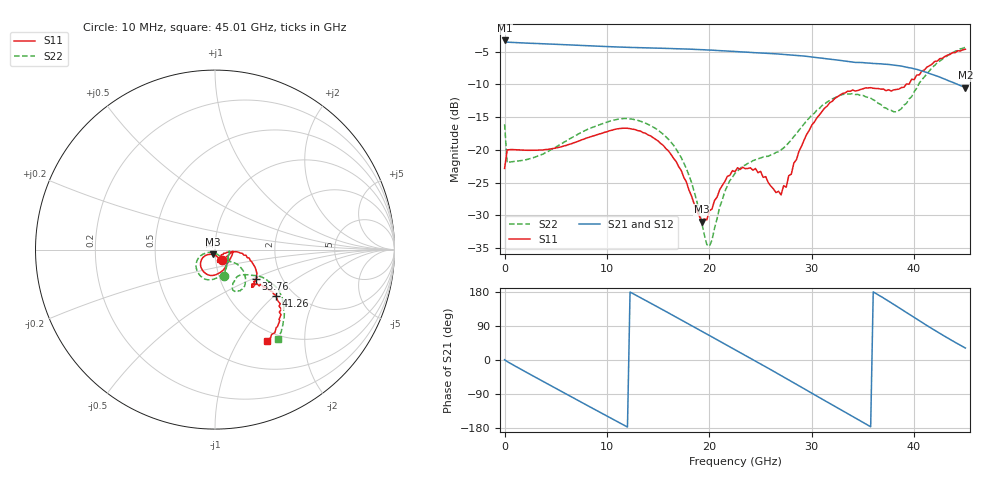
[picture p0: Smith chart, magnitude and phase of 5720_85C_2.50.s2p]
! Device:  ADRF5720
! Description: 0.5dB LSB GaAs MMIC 6-bit Digital Attenuator
! Frequency:  0.000009 -  40 GHz
! Ports:
!	RF1	= Port 1
!	RF2	= Port 2
! Vdd:  3.3 Volt
! Vss:  -3.3 Volt
! Control:  0/3.3 Volt
! State:  2.50 dB attenuation
! Data:  The device was measured using G-S-G Probes on a matrix board.
!  Data was collected using an calibrated 4 port network analyzer.
!  The reference plane for this measurement is at the launchers.
! Note:  Analog Devices supplies this data as a sample of measured data
!  for this product.  Your particular data for this product may vary.
!  Data was taken at 85 degrees C.
!  Analog Devices reserves the right to change this data at anytime.
# GHZ S DB R 45.0
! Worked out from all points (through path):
!   181 points, 10 MHz to 45.01 GHz, reference 45 ohm
!   highest |S21| = -3.30 dB at 10 MHz (marker M1); lowest = -10.5 dB at 45.01 GHz (marker M2)
!   group delay of S21, straight-line fit = 42.2 ps
!   lowest |S11| = -30.9 dB at 19.26 GHz (marker M3), VSWR 1.06, Z = 44 - j2.34 ohm
!   |S11| at or under -10 dB: start of sweep to 39.23 GHz
!   |S22| runs from -34.7 to -4.3 dB; largest |S21 - S12| = 0.0037
!   S11 on the Smith chart (normalised r, x): 10 MHz: 1.07, -0.13; 33.76 GHz: 1.47, -0.53; 41.26 GHz: 1.63, -1.03; 45.01 GHz: 0.86, -1.33
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0.01  -22.82 -57.0  -3.30 0.7  -3.28 0.7  -16.10 -71.0
0.26  -20.01 -5.7  -3.56 -4.0  -3.55 -4.0  -21.96 -5.8
2.01  -20.04 -21.1  -3.69 -30.6  -3.68 -30.5  -21.53 -19.7
4.26  -19.92 -42.8  -3.84 -63.8  -3.82 -63.8  -20.23 -42.6
7.76  -18.36 -66.3  -4.08 -115.2  -4.06 -115.1  -17.13 -70.4
11.51  -16.70 -99.5  -4.32 -169.7  -4.31 -169.6  -15.23 -104.3
13.26  -17.12 -117.1  -4.40 164.8  -4.39 165.0  -15.61 -121.2
15.26  -19.03 -135.9  -4.48 135.4  -4.47 135.6  -17.31 -140.5
17.76  -24.88 -146.6  -4.61 98.4  -4.59 98.6  -22.83 -159.2
19.26  -30.93 -110.6  -4.71 75.9  -4.69 76.1  -31.09 -146.7
20.01  -29.27 -84.7  -4.76 64.7  -4.74 64.9  -34.69 -100.8
21.51  -24.84 -66.5  -4.89 42.2  -4.88 42.4  -26.35 -53.4
22.76  -22.72 -70.7  -5.01 23.5  -4.99 23.7  -23.21 -54.5
24.76  -23.48 -77.8  -5.19 -6.7  -5.17 -6.4  -21.35 -57.0
27.01  -26.87 -39.3  -5.40 -41.0  -5.38 -40.7  -20.00 -41.6
30.26  -15.74 -10.8  -5.87 -91.5  -5.85 -91.2  -14.40 -36.2
33.76  -11.05 -36.0  -6.54 -145.4  -6.52 -145.0  -11.47 -56.8
35.76  -10.50 -44.4  -6.77 -176.3  -6.75 -175.9  -12.10 -66.0
37.76  -11.02 -42.7  -7.01 151.1  -7.00 151.4  -13.96 -54.7
38.76  -10.48 -40.7  -7.21 134.0  -7.19 134.4  -13.72 -42.6
41.26  -7.36 -37.0  -8.20 90.9  -8.18 91.3  -8.36 -30.9
45.01  -4.64 -60.5  -10.48 31.6  -10.45 32.0  -4.33 -54.9
